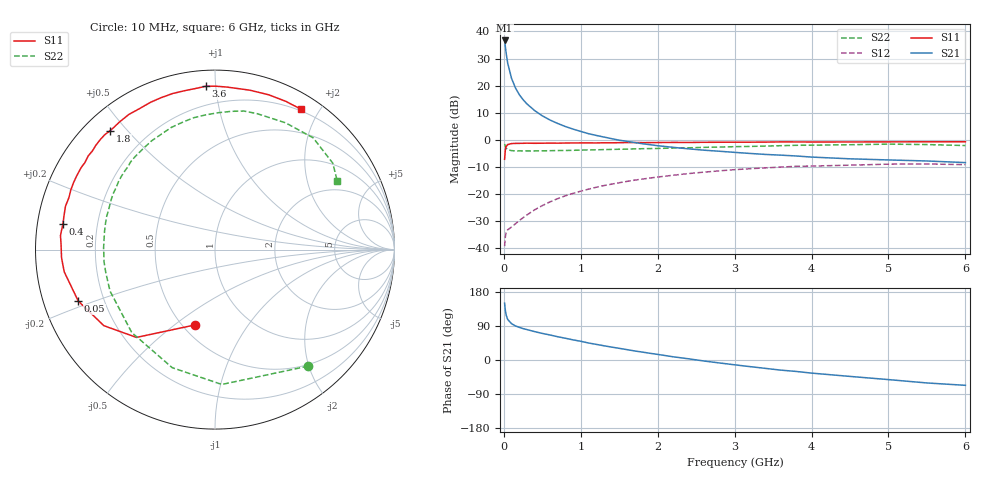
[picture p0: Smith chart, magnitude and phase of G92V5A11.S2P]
! SIEMENS Small Signal Semiconductors
! BFG235
! Si NPN RF Bipolar Junction Transistor in SOT223
! VCE = 2.5 V  IC = 110 mA
! Common Emitter S-Parameters:  July  1994
# GHz  S  MA  R  50
!  f  S11  S21  S12  S22
! GHz  MAG  ANG  MAG  ANG  MAG  ANG  MAG  ANG
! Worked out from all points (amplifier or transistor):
!   40 points, 10 MHz to 6 GHz, reference 50 ohm
!   highest |S21| = 36.7 dB at 10 MHz (marker M1)
!   |S21| within 3 dB of that: start of sweep to 22.66 MHz
!   unconditionally stable (mu >= 1): 451.3 MHz to 1.522 GHz
!   at 200 MHz: K = 0.79, MSG = 23.3 dB, |S12| = -29.9 dB
!   at 1.5 GHz: K = 1.00, MAG = 7.5 dB, |S12| = -15.9 dB
!   at 6 GHz: K = 0.92, MSG = 0.4 dB, |S12| = -9.2 dB
!   S11 on the Smith chart (normalised r, x): 10 MHz: 0.57, -0.59; 50 MHz: 0.11, -0.18; 400 MHz: 0.08, +0.08; 1.8 GHz: 0.07, +0.45; 3.6 GHz: 0.09, +0.94; 6 GHz: 0.18, +1.76
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0.01  0.4352 -105.1  68.24 149.9  0.0108 60.7  0.8308 -51.4
0.02  0.6562 -131.8  51.84 130.3  0.0163 45.4  0.7524 -87.1
0.03  0.7504 -145.6  39.78 118.8  0.0192 38.2  0.6997 -109.9
0.05  0.814 -159.4  26.05 107.0  0.0217 31.3  0.6547 -135.1
0.1  0.8491 -171.6  13.62 95.8  0.0244 34.5  0.6289 -158.5
0.15  0.8563 -177.0  9.129 90.0  0.0279 40.9  0.6218 -168.1
0.2  0.8566 180.0  6.827 86.3  0.0321 45.5  0.622 -173.6
0.25  0.8595 177.1  5.499 82.9  0.0362 49.2  0.6199 -177.5
0.3  0.8646 174.8  4.596 80.3  0.0407 52.1  0.6209 179.2
0.4  0.8592 170.4  3.458 74.9  0.0507 55.1  0.6209 174.4
0.5  0.8627 166.9  2.765 70.2  0.0606 56.5  0.6239 170.3
0.6  0.8673 163.8  2.313 66.0  0.0711 56.4  0.6273 166.5
0.7  0.8639 160.4  1.998 61.4  0.0816 56.1  0.6311 163.0
0.9  0.8718 154.8  1.571 53.1  0.1021 53.5  0.6371 156.7
1.1  0.8745 148.5  1.294 44.9  0.1221 50.1  0.6479 150.6
1.8  0.8833 131.4  0.844 20.9  0.1876 35.5  0.6828 130.9
2.2  0.8931 122.5  0.724 8.5  0.2207 26.5  0.7016 120.1
3.2  0.9012 101.2  0.558 -17.5  0.2914 3.3  0.752 94.1
3.6  0.9116 93.1  0.519 -26.7  0.3122 -6.6  0.7758 83.2
4.5  0.9091 77.6  0.444 -43.3  0.3389 -26.0  0.8084 60.9
5.5  0.9153 64.5  0.405 -60.6  0.3564 -47.5  0.814 36.3
6  0.9172 58.7  0.378 -66.8  0.3463 -55.7  0.7809 29.2
